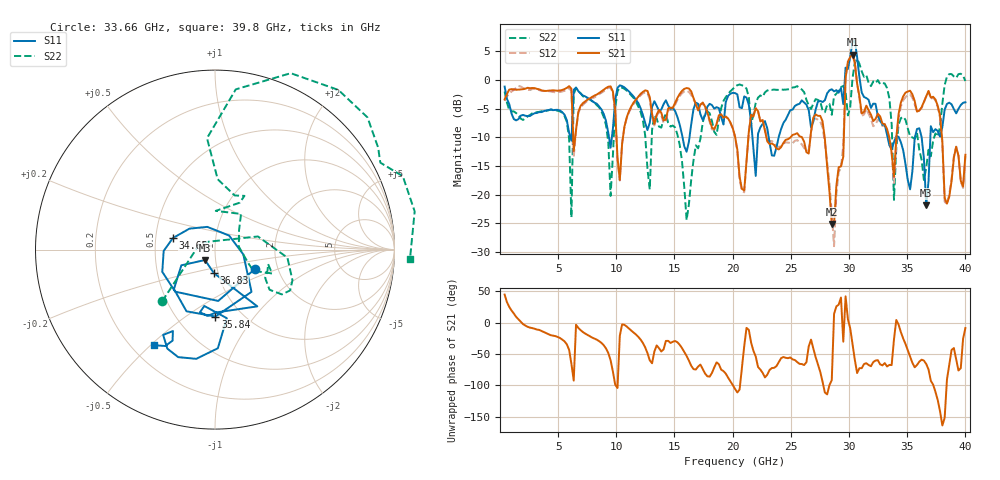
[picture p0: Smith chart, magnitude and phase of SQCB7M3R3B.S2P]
! Network Analyzer HP8722ES.07.66: Jul 25, 2000 Serial No. US39175408
! 26 Oct 2004  13:41:07
! Frequency  S11  S21  S12  S22
# HZ  S  DB R  50
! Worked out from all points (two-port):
!   201 points, 400 MHz to 40 GHz, reference 50 ohm
!   highest |S21| = 4.42 dB at 30.3 GHz (marker M1); lowest = -25.2 dB at 28.52 GHz (marker M2)
!   |S21| within 3 dB of the highest: 29.78 GHz to 30.58 GHz (800.5 MHz wide, 2.65 % of centre)
!   lowest |S11| = -21.9 dB at 36.63 GHz (marker M3), VSWR 1.17, Z = 44.4 - j5.19 ohm
!   |S11| at or under -10 dB: 15.69 GHz to 16.29 GHz (601.6 MHz wide, 3.76 % of centre); 23.1 GHz to 23.95 GHz (857.1 MHz wide, 3.64 % of centre); 34.27 GHz to 35.66 GHz (1.389 GHz wide, 3.97 % of centre)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
!   |S22| runs from -24.4 to 3.7 dB; largest |S21 - S12| = 0.11
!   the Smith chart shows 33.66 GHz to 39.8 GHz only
!   S11 on the Smith chart (normalised r, x): 33.66 GHz: 1.53, -0.35; 34.65 GHz: 0.62, +0.08; 35.84 GHz: 0.76, -0.66; 36.83 GHz: 0.95, -0.25; 39.8 GHz: 0.29, -0.51
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4e8  -1.16 -46.9  -3.41 44.7  -3.64 49.9  -2.03 -38.5
6.142e9  -10.59 -45.9  -1.53 -65.7  -1.92 -67.0  -23.99 28.0
7.132e9  -2.72 -89.8  -4.04 -15.1  -4.34 -17.1  -2.85 -119.3
1.3666e10  -5.39 -50.0  -5.22 -40.6  -5.58 -40.9  -8.14 -102.6
2.02e10  -2.30 -20.8  -9.82 -105.4  -9.91 -106.0  -1.19 -22.9
2.6932e10  -7.27 89.5  -6.57 -41.3  -6.83 -46.8  -4.13 -32.6
2.8516e10  -1.63 16.6  -25.15 -91.7  -23.24 -98.4  -6.09 -9.5
2.9506e10  -4.21 18.4  -13.40 -30.4  -11.37 -22.6  -1.04 39.1
2.9704e10  2.13 -54.2  0.33 41.8  0.64 36.3  -2.10 -93.5
3.0298e10  6.62 -125.4  4.42 -34.3  4.34 -34.4  0.27 3.0
3.0496e10  6.88 -156.5  2.93 -59.0  3.30 -60.2  2.96 -16.4
3.0694e10  3.97 -18.0  -0.64 -80.3  -0.67 -85.0  3.67 142.3
3.1288e10  -2.98 -33.3  -5.58 -65.9  -6.03 -70.0  0.54 124.6
3.1486e10  -3.17 153.8  -4.48 -64.6  -5.12 -67.8  0.82 -56.0
3.3466e10  -11.39 38.4  -10.11 -67.3  -10.33 -68.3  -3.23 -109.1
3.3664e10  -12.12 -25.7  -12.74 -67.6  -12.86 -71.3  -7.70 -135.6
3.4654e10  -12.28 164.7  -2.87 -25.3  -3.55 -22.8  -6.44 -28.6
3.5842e10  -8.57 -89.6  -5.53 -67.4  -5.58 -63.2  -9.25 -22.7
3.6634e10  -21.89 -133.9  -2.85 -65.9  -2.87 -63.7  -15.32 38.7
3.6832e10  -17.68 -92.9  -1.92 -74.6  -2.01 -73.0  -12.18 53.9
3.9802e10  -3.99 -122.5  -18.56 -25.7  -18.84 -23.7  0.73 -2.9
4e10  -3.90 -126.8  -13.06 -8.6  -13.34 -6.6  -0.19 -15.5
